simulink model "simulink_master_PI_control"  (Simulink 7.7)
settings: Solver=ode23tb  StartTime=0.0  StopTime=54000  RelTol=1e-3
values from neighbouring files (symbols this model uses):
  Tf_set = 292    [model_master_simulink_floor.m]    (also in model_master_simulink_PI_tuning.m = 293; model_master_simulink_storing_floorroom.m = 293)
  To = 273+0    (= 273)    [model_master_simulink_floor.m]    (also in model_master_simulink_PI_tuning.m; model_master_simulink_storing_floorroom.m; sfunctionmodel.m = u(3); equations.m = d(1))
  Tr_set = 292    [model_master_simulink_floor.m]    (also in model_master_simulink_PI_tuning.m; model_master_simulink_storing_floorroom.m)
libraries: simulink x2

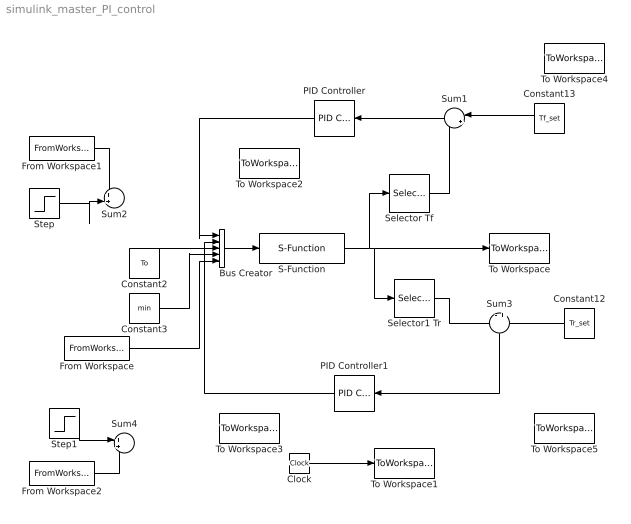
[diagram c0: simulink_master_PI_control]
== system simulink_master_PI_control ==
  Bus Creator : BusCreator  Inputs=5
  Clock : Clock
  Constant12 : Constant  Value=Tr_set
  Constant13 : Constant  Value=Tf_set
  Constant2 : Constant  Value=To
  Constant3 : Constant  Value=min
  From Workspace : FromWorkspace  VariableName=var  SampleTime=0  Interpolate=off  OutputAfterFinalValue=Holding final value
  From Workspace1 : FromWorkspace  VariableName=varqhf  SampleTime=0
  From Workspace2 : FromWorkspace  VariableName=varqhr  SampleTime=0
  PID Controller : simulink/Continuous/PID Controller  SystemSampleTime=-1  Controller=PI  TimeDomain=Continuous-time  SampleTime=1  IntegratorMethod=Forward Euler  FilterMethod=Forward Euler  Form=Parallel  P=127.7  I=3192.5*0.0001  D=0  N=100  InitialConditionSource=internal  InitialConditionForIntegrator=0  InitialConditionForFilter=0  ExternalReset=none  LimitOutput=on  UpperSaturationLimit=2.5  LowerSaturationLimit=0  LinearizeAsGain=off  AntiWindupMode=clamping  Kb=1  TrackingMode=off  Kt=1  PParamMin=[]  PParamMax=[]  IParamMin=[]  IParamMax=[]  DParamMin=[]  DParamMax=[]  NParamMin=[]  NParamMax=[]  KbParamMin=[]  KbParamMax=[]  KtParamMin=[]  KtParamMax=[]  POutMin=[]  POutMax=[]  IOutMin=[]  IOutMax=[]  DOutMin=[]  DOutMax=[]  NOutMin=[]  NOutMax=[]  KbOutMin=[]  KbOutMax=[]  KtOutMin=[]  KtOutMax=[]  IntegratorOutMin=[]  IntegratorOutMax=[]  FilterOutMin=[]  FilterOutMax=[]  SumOutMin=[]  SumOutMax=[]  SumI1OutMin=[]  SumI1OutMax=[]  SumI2OutMin=[]  SumI2OutMax=[]  SumI3OutMin=[]  SumI3OutMax=[]  SumDOutMin=[]  SumDOutMax=[]  SaturationOutMin=[]  SaturationOutMax=[]  IntegratorContinuousStateAttributes=''  IntegratorStateMustResolveToSignalObject=off  IntegratorRTWStateStorageClass=Auto  FilterContinuousStateAttributes=''  FilterStateMustResolveToSignalObject=off  FilterRTWStateStorageClass=Auto
  PID Controller1 : simulink/Continuous/PID Controller  SystemSampleTime=-1  Controller=PI  TimeDomain=Continuous-time  SampleTime=1  IntegratorMethod=Forward Euler  FilterMethod=Forward Euler  Form=Parallel  P=249.7  I=6242.5*0.1  D=0  N=100  InitialConditionSource=internal  InitialConditionForIntegrator=0  InitialConditionForFilter=0  ExternalReset=none  LimitOutput=on  UpperSaturationLimit=2  LowerSaturationLimit=0  LinearizeAsGain=off  AntiWindupMode=clamping  Kb=1  TrackingMode=off  Kt=1  PParamMin=[]  PParamMax=[]  IParamMin=[]  IParamMax=[]  DParamMin=[]  DParamMax=[]  NParamMin=[]  NParamMax=[]  KbParamMin=[]  KbParamMax=[]  KtParamMin=[]  KtParamMax=[]  POutMin=[]  POutMax=[]  IOutMin=[]  IOutMax=[]  DOutMin=[]  DOutMax=[]  NOutMin=[]  NOutMax=[]  KbOutMin=[]  KbOutMax=[]  KtOutMin=[]  KtOutMax=[]  IntegratorOutMin=[]  IntegratorOutMax=[]  FilterOutMin=[]  FilterOutMax=[]  SumOutMin=[]  SumOutMax=[]  SumI1OutMin=[]  SumI1OutMax=[]  SumI2OutMin=[]  SumI2OutMax=[]  SumI3OutMin=[]  SumI3OutMax=[]  SumDOutMin=[]  SumDOutMax=[]  SaturationOutMin=[]  SaturationOutMax=[]  IntegratorContinuousStateAttributes=''  IntegratorStateMustResolveToSignalObject=off  IntegratorRTWStateStorageClass=Auto  FilterContinuousStateAttributes=''  FilterStateMustResolveToSignalObject=off  FilterRTWStateStorageClass=Auto
  S-Function : S-Function  FunctionName=sfunctionmodel  Parameters=init, par,var  EnableBusSupport=off
  Selector Tf : Selector  InputPortWidth=3  IndexOptions=Index vector (dialog)  Indices=1  OutputSizes=1
  Selector1 Tr : Selector  InputPortWidth=3  IndexOptions=Index vector (dialog)  Indices=2  OutputSizes=1
  Step : Step  Time=10*60*60  After=5  SampleTime=0
  Step1 : Step  Time=10*60*60  After=4  SampleTime=0
  Sum1 : Sum  Inputs=|+-
  Sum2 : Sum
  Sum3 : Sum  Inputs=-+
  Sum4 : Sum
  To Workspace : ToWorkspace  VariableName=simout  SampleTime=-1  SaveFormat=Array
  To Workspace1 : ToWorkspace  VariableName=time  SampleTime=-1  SaveFormat=Array
  To Workspace2 : ToWorkspace  VariableName=qhf_out  SampleTime=-1  SaveFormat=Array
  To Workspace3 : ToWorkspace  VariableName=qhr_out  SampleTime=-1  SaveFormat=Array
  To Workspace4 : ToWorkspace  VariableName=Tf_set_out  SampleTime=-1  SaveFormat=Array
  To Workspace5 : ToWorkspace  VariableName=Tr_set_out  SampleTime=-1  SaveFormat=Array
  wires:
  Constant3/1 -> Bus Creator/4
  Bus Creator/1 -> S-Function/1
  S-Function/1 -> Selector Tf/1, To Workspace/1, Selector1 Tr/1
  Clock/1 -> To Workspace1/1
  Selector1 Tr/1 -> Sum3/1
  Sum3/1 -> PID Controller1/1
  Constant2/1 -> Bus Creator/3
  Selector Tf/1 -> Sum1/2
  Sum1/1 -> PID Controller/1
  From Workspace/1 -> Bus Creator/5
  Step/1 -> Sum2/2
  Constant13/1 -> Sum1/1
  Constant12/1 -> Sum3/2
  From Workspace1/1 -> Sum2/1
  PID Controller/1 -> Bus Creator/1
  PID Controller1/1 -> Bus Creator/2
  Step1/1 -> Sum4/1
  From Workspace2/1 -> Sum4/2
